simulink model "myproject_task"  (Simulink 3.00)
libraries: mathlib x11, arclib x4, modellib x2

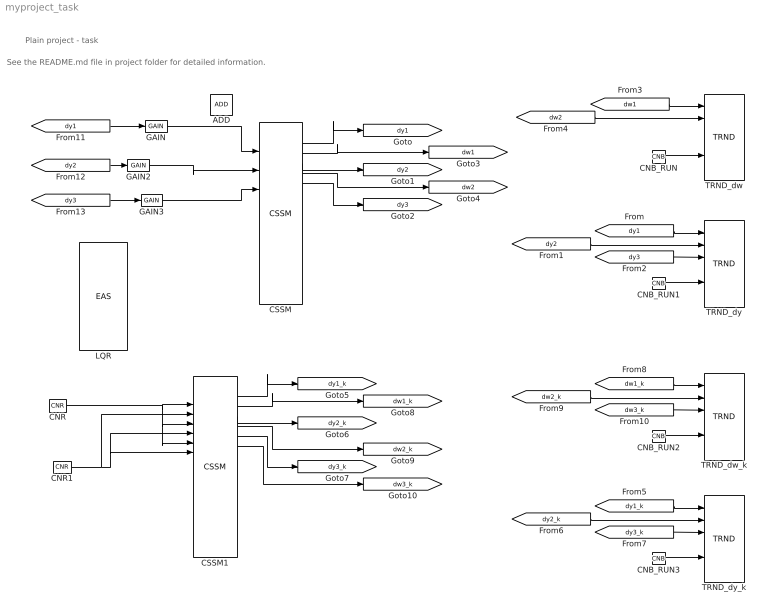
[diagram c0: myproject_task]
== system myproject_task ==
  note: Plain project - task
  note: See the README.md file in project folder for detailed information.
  ADD : mathlib/ADD
  CNB_RUN{,1..3} (4 alike) : mathlib/CNB  YCN=on
  CNR : mathlib/CNR  ycn=1
  CNR1 : mathlib/CNR  ycn=1
  CSSM : modellib/CSSM  UD=off  is=2  eps=1E-15  Ac=[ -1 0 0 0 0; 1 0 -1 0 0; 0 0 -2 0 0; 0 0 1 0 -1; 0 0 0 0 -1]  Bc=[1 0 0; 0 0 0; 0 1 0; 0 0 0; 0 0 1]  Cc=[ 1 0 0 0 0; 0 1 0 0 0; 0 0 1 0 0; 0 0 0 1 0; 0 0 0 0 1]  Dc=[ 0 0 0; 0 0 0; 0 0 0; 0 0 0; 0 0 0]  x0=[ 0; 0; 0; 0; 0]
  CSSM1 : modellib/CSSM  UD=off  is=2  eps=1E-15  Ac=[ -1 0 0 0 0 0; 1 0 -1 0 0 0; 0 0 -2 0 0 0; 0 0 1 0 -1 0; 0 0 0 0 -1 0; -1 0 0 0 1 0]  Bc=[ 1 0 0; 0 0 0; 0 1 0; 0 0 0; 0 0 1; 0 0 0]  Cc=[ 1 0 0 0 0 0; 0 1 0 0 0 0; 0 0 1 0 0 0; 0 0 0 1 0 0; 0 0 0 0 1 0; 0 0 0 0 0 1]  Dc=[ 0 0 0; 0 0 0; 0 0 0; 0 0 0; 0 0 0; 0 0 0]  x0=[ 0; 0; 0; 0; 0; 0]
  GAIN : mathlib/GAIN  k=-1
  GAIN2 : mathlib/GAIN  k=-1
  GAIN3 : mathlib/GAIN  k=-1
  LQR : mathlib/EAS  a=1  b=1  c=1  d=1  y0=0
  TRND_dw : arclib/TRND  n=2  l=100000  btype=8  ptype1=1: Store  ptype2=1: Store  ptype3=1: Store  ptype4=1: Store  pfac=1  afac=0  arc=0  id=1  Title=Trend Title  timesrc=1
  TRND_dw_k : arclib/TRND  n=3  l=100000  btype=8  ptype1=1: Store  ptype2=1: Store  ptype3=1: Store  ptype4=1: Store  pfac=1  afac=0  arc=0  id=1  Title=Trend Title  timesrc=1
  TRND_dy : arclib/TRND  n=3  l=100000  btype=8  ptype1=1: Store  ptype2=1: Store  ptype3=1: Store  ptype4=1: Store  pfac=1  afac=0  arc=0  id=1  Title=Trend Title  timesrc=1
  TRND_dy_k : arclib/TRND  n=3  l=100000  btype=8  ptype1=1: Store  ptype2=1: Store  ptype3=1: Store  ptype4=1: Store  pfac=1  afac=0  arc=0  id=1  Title=Trend Title  timesrc=1
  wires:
  CNB_RUN/1 -> TRND_dw/5
  CNB_RUN1/1 -> TRND_dy/5
  CNB_RUN2/1 -> TRND_dw_k/5
  CNB_RUN3/1 -> TRND_dy_k/5
  CNR/1 -> CSSM1/3, CSSM1/5, CSSM1/7
  CNR1/1 -> CSSM1/4, CSSM1/6, CSSM1/8
  CSSM/2 -> [dy1]
  CSSM/3 -> [dw1]
  CSSM/4 -> [dy2]
  CSSM/5 -> [dw2]
  CSSM/6 -> [dy3]
  CSSM1/2 -> [dy1_k]
  CSSM1/3 -> [dw1_k]
  CSSM1/4 -> [dy2_k]
  CSSM1/5 -> [dw2_k]
  CSSM1/6 -> [dy3_k]
  CSSM1/7 -> [dw3_k]
  [dy1] -> TRND_dy/1
  [dy2] -> TRND_dy/2
  [dw3_k] -> TRND_dw_k/3
  [dy1] -> GAIN/1
  [dy2] -> GAIN2/1
  [dy3] -> GAIN3/1
  [dy3] -> TRND_dy/3
  [dw1] -> TRND_dw/1
  [dw2] -> TRND_dw/2
  [dy1_k] -> TRND_dy_k/1
  [dy2_k] -> TRND_dy_k/2
  [dy3_k] -> TRND_dy_k/3
  [dw1_k] -> TRND_dw_k/1
  [dw2_k] -> TRND_dw_k/2
  GAIN/1 -> CSSM/3
  GAIN2/1 -> CSSM/5
  GAIN3/1 -> CSSM/7
